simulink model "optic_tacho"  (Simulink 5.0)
settings: Solver=ode4  StartTime=0.0  StopTime=4  FixedStep=0.001  RelTol=1e-3
libraries: simulink x1

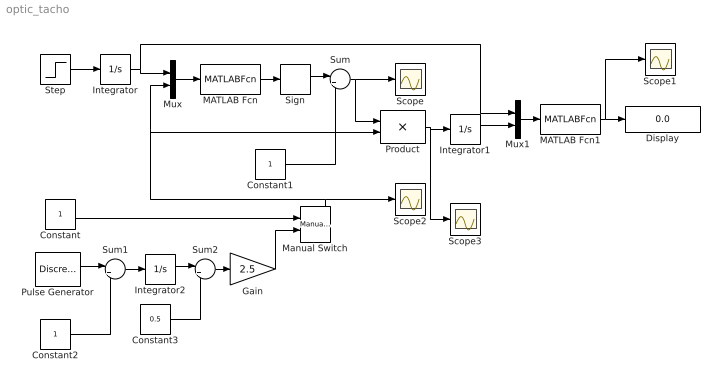
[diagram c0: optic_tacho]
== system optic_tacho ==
  Constant : Constant
  Constant1 : Constant
  Constant2 : Constant
  Constant3 : Constant  Value=0.5
  Display : Display
  Gain : Gain  Gain=2.5
  Integrator : Integrator
  Integrator1 : Integrator
  Integrator2 : Integrator
  MATLAB Fcn : MATLABFcn  MATLABFcn=v2f
  MATLAB Fcn1 : MATLABFcn  MATLABFcn=perata
  Manual Switch : simulink/Signal Routing/Manual Switch  sw=0  action=0
  Mux : Mux  Inputs=2
  Mux1 : Mux  Inputs=2
  Product : Product
  Pulse Generator : DiscretePulseGenerator  PulseType=Time based  Amplitude=2  PulseWidth=50
  Scope{,1..3} (4 alike) : Scope
  Sign : Signum
  Step : Step  Time=0  SampleTime=0
  Sum : Sum  Inputs=|++
  Sum1 : Sum  Inputs=|+-
  Sum2 : Sum  Inputs=|+-
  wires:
  Step/1 -> Integrator/1
  Integrator/1 -> Mux/1, Mux1/1
  Mux/1 -> MATLAB Fcn/1
  MATLAB Fcn/1 -> Sign/1
  Product/1 -> Integrator1/1, Scope3/1
  Integrator1/1 -> Mux1/2
  Mux1/1 -> MATLAB Fcn1/1
  MATLAB Fcn1/1 -> Display/1, Scope1/1
  Sign/1 -> Sum/1
  Sum/1 -> Scope/1, Product/1
  Pulse Generator/1 -> Sum1/1
  Constant2/1 -> Sum1/2
  Sum1/1 -> Integrator2/1
  Integrator2/1 -> Sum2/1
  Constant3/1 -> Sum2/2
  Sum2/1 -> Gain/1
  Gain/1 -> Manual Switch/2
  Constant1/1 -> Sum/2
  Manual Switch/1 -> Mux/2, Product/2, Scope2/1
  Constant/1 -> Manual Switch/1
